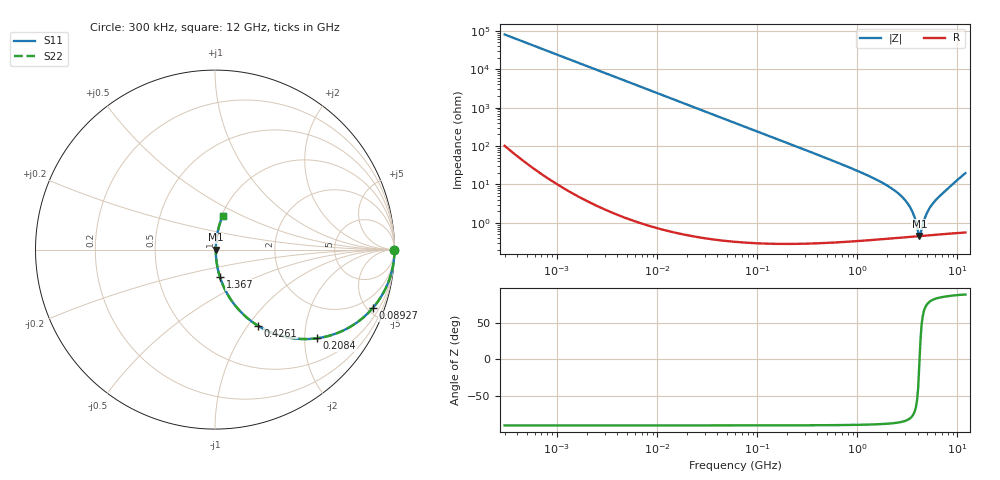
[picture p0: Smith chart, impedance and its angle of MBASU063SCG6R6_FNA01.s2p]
! MBASU063SCG6R6_FNA01  S-PARAMETER MODEL  ( General Type )
! Model Generated by TAIYO YUDEN Corporation (http://www.ty-top.com)
! Version 1.0
! TAIYO YUDEN Control No. 130801
! Copyright(c) 2013 TAIYO YUDEN CO.,LTD. All Rights Reserved.
! Product Description (link to TY-COMPAS)
! https://ds.yuden.co.jp/TYCOMPAS/or/detail?pn=MBASU063SCG6R6DFNA01&u=M
! Products Name : Multilayer Ceramic Capacitors
! Characteristics :
!  Capacitance : 6.6 pF , Rated Voltage : 50V , TCC : CG / C0G
!  Case Size : 0.6 x 0.3 / 0.024 x 0.012 [mm/inch] , Thickness : 0.3 / 0.012 [mm/inch]
!  (Conditions: Temperature = 25 degC , DC Bias Current/Voltage = 0A / 0V)
! External Node Assignments :
!  1  o---| |---o  2
! GND o---------o GND
! Frequency Range : 0.3MHz  -  12000MHz  [ 401 STEP ]
# MHz S RI R 50
! Freq[MHz].  S11 Real  S11 Imag  S21 Real  S21 Imag  S12 Real  S12 Imag  S22 Real  S22 Imag
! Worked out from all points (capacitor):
!   401 points, 300 kHz to 12 GHz, reference 50 ohm
!   read as one part in series: C = 6.62 pF near 316.3 kHz
!   lowest |Z| = 459 mohm at 4.159 GHz (marker M1)
!   series resonance near 4.184 GHz, so ESL is about 220 pH
!   S11 on the Smith chart (normalised r, x): 300 kHz: open; 89.27 MHz: 1.01, -5.39; 208.4 MHz: 1.01, -2.30; 426.1 MHz: 1.01, -1.12; 1.367 GHz: 1.01, -0.31; 12 GHz: 1.01, +0.39
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0.3  1 -0.00125  3.13e-06 0.00125  3.13e-06 0.00125  1 -0.00125
1.769972  0.9999 -0.00736  5.65e-05 0.00736  5.65e-05 0.00736  0.9999 -0.00736
10.44266  0.9981 -0.0433  0.00189 0.0433  0.00189 0.0433  0.9981 -0.0433
27.10171  0.9874 -0.1113  0.0126 0.1113  0.0126 0.1113  0.9874 -0.1113
60  0.9412 -0.2348  0.0588 0.2348  0.0588 0.2348  0.9412 -0.2348
89.27472  0.8785 -0.3261  0.1215 0.3261  0.1215 0.3261  0.8785 -0.3261
208.3979  0.5698 -0.4939  0.4302 0.4939  0.4302 0.4939  0.5698 -0.4939
353.9943  0.3135 -0.4618  0.6865 0.4618  0.6865 0.4618  0.3135 -0.4618
426.1204  0.239 -0.4238  0.761 0.4238  0.761 0.4238  0.239 -0.4238
723.8279  0.0964 -0.2903  0.9036 0.2903  0.9036 0.2903  0.0964 -0.2903
1366.97  0.0274 -0.1523  0.9726 0.1523  0.9726 0.1523  0.0274 -0.1523
2088.533  0.0112 -0.0851  0.9888 0.0851  0.9888 0.0851  0.0112 -0.0851
2650.866  0.00699 -0.0537  0.993 0.0537  0.993 0.0537  0.00699 -0.0537
3190.978  0.00524 -0.0312  0.9948 0.0312  0.9948 0.0312  0.00524 -0.0312
3547.679  0.00472 -0.0188  0.9953 0.0188  0.9953 0.0188  0.00472 -0.0188
4050.141  0.00451 -0.00363  0.9955 0.00363  0.9955 0.00363  0.00451 -0.00363
4158.869  0.00452 -0.000631  0.9955 0.000631  0.9955 0.000631  0.00452 -0.000631
4385.161  0.0046 0.00506  0.9954 -0.00506  0.9954 -0.00506  0.0046 0.00506
5006.236  0.00505 0.0184  0.995 -0.0184  0.995 -0.0184  0.00505 0.0184
5715.274  0.00588 0.0322  0.9941 -0.0322  0.9941 -0.0322  0.00588 0.0322
8281.503  0.0122 0.083  0.9878 -0.083  0.9878 -0.083  0.0122 0.083
12000  0.0423 0.1875  0.9577 -0.1875  0.9577 -0.1875  0.0423 0.1875
